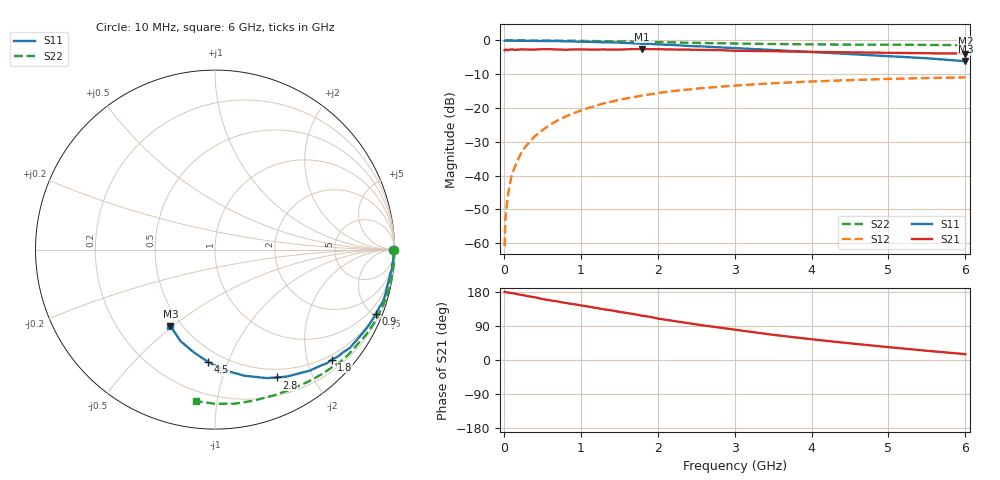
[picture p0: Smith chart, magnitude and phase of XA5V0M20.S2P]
! SIEMENS Discrete & RF Semiconductors
! BFY180
! Si NPN RF Bipolar Junction Transistor in MICRO-X
! VCE = 5 V  IC = 0.2 mA
! Common Emitter S-Parameters:  May  1997
# GHz  S  MA  R  50
!  f  S11  S21  S12  S22
! GHz  MAG  ANG  MAG  ANG  MAG  ANG  MAG  ANG
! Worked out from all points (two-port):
!   36 points, 10 MHz to 6 GHz, reference 50 ohm
!   highest |S21| = -2.52 dB at 1.8 GHz (marker M1); lowest = -3.9 dB at 6 GHz (marker M2)
!   |S21| within 3 dB of the highest: start of sweep to end of sweep
!   lowest |S11| = -6.2 dB at 6 GHz (marker M3), VSWR 2.94, Z = 21.8 - j24.4 ohm
!   |S11| at or under -10 dB: nowhere
!   |S22| runs from -1.4 to 0.0 dB; largest |S21 - S12| = 0.74
!   S11 on the Smith chart (normalised r, x): 10 MHz: open; 900 MHz: 0.49, -5.15; 1.8 GHz: 0.40, -2.46; 2.8 GHz: 0.40, -1.52; 4.5 GHz: 0.41, -0.85; 6 GHz: 0.44, -0.49
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0.01  0.9919 -0.1  0.716 179.9  0.0009 87.0  0.9992 -0.2
0.02  0.9974 -0.5  0.733 179.0  0.0023 91.7  0.9999 -0.4
0.05  0.9946 -1.1  0.72 178.3  0.0049 86.7  0.9994 -1.0
0.1  0.9949 -2.6  0.738 176.7  0.01 89.4  0.9981 -2.0
0.2  0.9903 -4.8  0.734 172.6  0.0189 85.3  0.9999 -4.0
0.25  0.9921 -6.3  0.738 171.2  0.0239 85.9  0.9999 -4.9
0.3  0.9876 -7.3  0.734 168.8  0.0285 84.0  0.9981 -5.9
0.4  0.9843 -9.6  0.732 165.5  0.0378 81.8  0.9975 -7.9
0.5  0.9799 -12.2  0.744 161.1  0.0469 79.5  0.9963 -9.9
0.7  0.98 -17.2  0.735 154.5  0.0655 75.3  0.9917 -13.9
0.9  0.9652 -21.8  0.735 147.5  0.0832 70.8  0.9878 -17.7
1.1  0.9545 -26.4  0.734 140.8  0.1 66.8  0.9804 -21.6
1.5  0.9298 -36.1  0.731 127.1  0.132 58.3  0.9667 -29.2
1.8  0.8943 -43.3  0.748 116.7  0.1529 52.7  0.9514 -34.7
2.2  0.8568 -51.9  0.735 103.3  0.1784 44.9  0.9375 -41.9
2.4  0.8294 -56.7  0.731 97.1  0.1877 41.4  0.9243 -45.2
2.8  0.7906 -64.3  0.72 85.6  0.2065 35.0  0.9086 -51.4
3.5  0.7214 -76.9  0.693 66.5  0.2328 24.9  0.887 -61.5
4  0.6742 -85.4  0.677 54.7  0.2468 18.2  0.8748 -68.6
4.5  0.6278 -93.4  0.667 44.0  0.2585 12.2  0.8686 -75.7
5.5  0.5449 -110.7  0.646 24.4  0.2777 0.5  0.8593 -90.0
6  0.4923 -120.3  0.64 15.4  0.2837 -5.5  0.8509 -97.2
